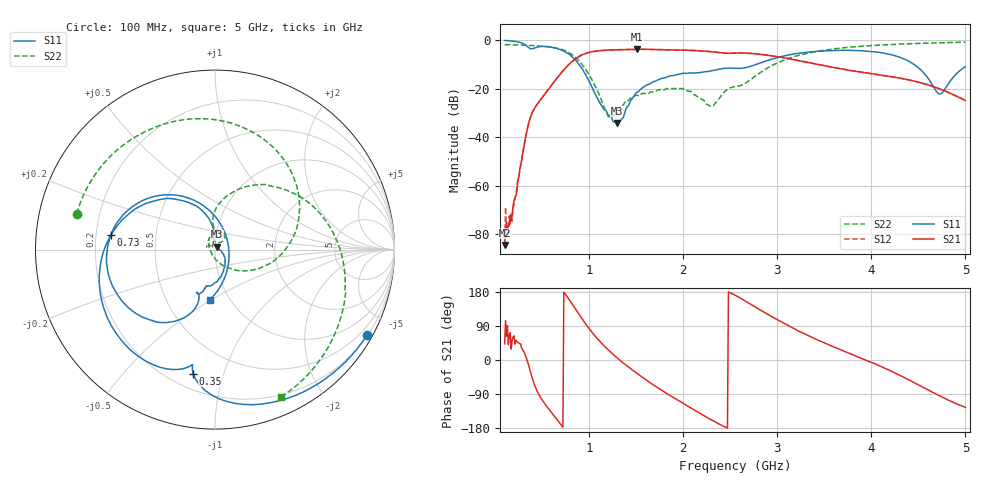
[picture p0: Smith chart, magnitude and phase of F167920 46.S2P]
!  2-Port S-parameters saved by WinCal
! VAR MeasName=S-Parameters (CALIBRATED_DATA) read from VNA (N5242A)
! VAR MeasDate=2016-11-22 9:57:46
! VAR NAME=F167920 46
! VAR FILENAME=F167920 46.S2P
! VAR DATE=2016-11-22 9:57:46
! VAR PHYS_PORTS=1,2
# Hz S DB R 50
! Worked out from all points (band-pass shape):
!   491 points, 100 MHz to 5 GHz, reference 50 ohm
!   highest |S21| = -3.86 dB at 1.51 GHz (marker M1); lowest = -84.3 dB at 100 MHz (marker M2)
!   |S21| within 3 dB of the highest: 890.3 MHz to 2.989 GHz (2.099 GHz wide, 108 % of centre)
!   lowest |S11| = -34.2 dB at 1.29 GHz (marker M3), VSWR 1.04, Z = 51 + j1.72 ohm
!   |S11| at or under -10 dB: 890.2 MHz to 2.781 GHz (1.891 GHz wide, 103 % of centre); 4.449 GHz to end of sweep
!   |S22| runs from -31.6 to -0.9 dB; largest |S21 - S12| = 0.0022
!   S11 on the Smith chart (normalised r, x): 100 MHz: 0.22, -3.82; 350 MHz: 0.29, -0.80; 730 MHz: 0.26, +0.07; 5 GHz: 0.81, -0.49
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1e8  -0.25 -29.3  -84.35 42.6  -84.82 25.2  -1.98 165.5
1.8e8  -0.51 -52.3  -72.08 51.4  -74.56 31.6  -2.04 153.8
2.7e8  -1.12 -79.2  -51.47 42.4  -51.86 38.5  -2.13 140.2
3.5e8  -3.08 -100.0  -35.23 -9.4  -35.17 -9.7  -2.26 127.4
5.1e8  -2.71 -125.3  -23.18 -109.2  -23.17 -109.2  -2.63 99.3
7.3e8  -4.65 172.0  -12.33 179.2  -12.32 179.1  -4.26 47.2
9.2e8  -11.54 113.1  -6.22 110.4  -6.22 110.4  -9.93 -13.8
1.04e9  -20.43 93.5  -4.80 69.8  -4.81 69.8  -17.26 -50.5
1.2e9  -30.86 102.6  -4.19 27.1  -4.19 27.1  -31.49 -135.7
1.29e9  -34.17 59.5  -4.08 7.0  -4.08 7.0  -29.18 157.2
1.51e9  -21.46 -48.9  -3.86 -35.7  -3.87 -35.8  -22.81 112.6
1.74e9  -16.27 -77.8  -4.01 -74.9  -4.01 -75.0  -20.59 92.0
1.99e9  -13.81 -96.7  -4.26 -112.7  -4.25 -112.7  -20.00 61.7
2.3e9  -12.75 -105.4  -4.88 -158.3  -4.87 -158.3  -27.42 74.6
2.55e9  -11.71 -113.5  -5.48 171.2  -5.47 171.2  -19.28 89.0
2.93e9  -8.07 -112.2  -6.50 116.0  -6.48 116.0  -10.82 80.4
3.37e9  -4.88 -142.4  -9.66 59.4  -9.61 59.2  -5.11 32.7
3.8e9  -4.34 -175.0  -12.72 14.1  -12.70 13.8  -2.92 -4.5
4.19e9  -5.92 149.8  -15.00 -26.9  -15.02 -27.2  -1.95 -29.0
4.49e9  -11.14 109.2  -17.25 -64.0  -17.29 -64.2  -1.49 -44.4
4.72e9  -22.22 14.9  -20.07 -93.9  -20.08 -93.9  -1.20 -54.5
5e9  -11.01 -96.1  -24.95 -125.0  -24.95 -125.1  -0.93 -65.7
